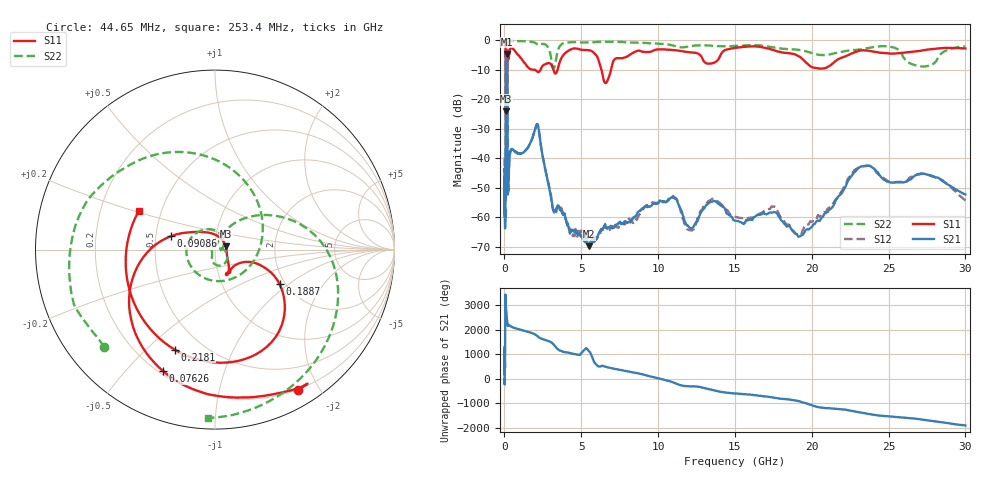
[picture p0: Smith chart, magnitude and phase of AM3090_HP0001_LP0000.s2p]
! Date/Time: Thu, Feb 28, 2019 1:53 PM
! Network Analyzer: Agilent Technologies E8364B Rev: A.07.50.67
! Sweep from 0.010 to 30.000 GHz, 1601 Points, Sweep Type: LOG
! Power Supply: 5.023 V, 0.002 A
# Hz S DB R 50
!freq MagS11 AngS11 MagS21 AngS21 MagS12 AngS12 MagS22 AngS22
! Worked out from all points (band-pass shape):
!   1601 points, 10 MHz to 30 GHz, reference 50 ohm
!   highest |S21| = -4.73 dB at 134.2 MHz (marker M1); lowest = -69.9 dB at 5.501 GHz (marker M2)
!   |S21| within 3 dB of the highest: 98.46 MHz to 174.1 MHz (75.63 MHz wide, 55.5 % of centre)
!   lowest |S11| = -24.1 dB at 98.44 MHz (marker M3), VSWR 1.13, Z = 56.3 + j2 ohm
!   |S11| at or under -10 dB: 1.806 GHz to 2.35 GHz (544.7 MHz wide, 26.2 % of centre); 3.182 GHz to 3.46 GHz (278.2 MHz wide, 8.38 % of centre); 6.308 GHz to 6.937 GHz (628.7 MHz wide, 9.49 % of centre)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
!   |S22| runs from -36.2 to -0.1 dB; largest |S21 - S12| = 0.013
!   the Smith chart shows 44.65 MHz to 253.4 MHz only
!   S11 on the Smith chart (normalised r, x): 44.65 MHz: 0.19, -1.73; 76.26 MHz: 0.22, -0.64; 90.86 MHz: 0.60, +0.10; 188.7 MHz: 1.86, -0.87; 218.1 MHz: 0.35, -0.61; 253.4 MHz: 0.37, +0.21
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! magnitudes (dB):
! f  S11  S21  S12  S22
! 10 MHz  -0.2  -44.5  -39.8  -0.5
! 38.04 MHz  -0.5  -60.0  -59.1  -1.3
! 44.65 MHz  -0.8  -56.7  -58.5  -1.7
! 76.26 MHz  -2.7  -42.9  -43.3  -5.2
! 90.86 MHz  -11.8  -14.0  -14.0  -15.2
! 98.44 MHz  -24.1  -7.7  -7.7  -16.6
! 134.2 MHz  -16.6  -4.7  -4.7  -29.8
! 144.7 MHz  -16.3  -4.9  -4.9  -21.2
! 169.8 MHz  -15.2  -6.8  -6.8  -36.1
! 188.7 MHz  -7.8  -17.8  -17.7  -10.7
! 218.1 MHz  -4.4  -52.3  -51.5  -1.5
! 253.4 MHz  -6.5  -50.7  -50.2  -0.6
! 550.5 MHz  -3.0  -37.2  -37.1  -0.2
! 2.084 GHz  -10.5  -28.8  -28.7  -1.2
! 3.236 GHz  -10.9  -58.1  -58.5  -9.4
! 5.501 GHz  -3.5  -69.9  -67.4  -0.8
! 6.619 GHz  -14.5  -63.5  -63.3  -0.6
! 7.926 GHz  -5.7  -61.6  -60.8  -0.8
! 10.81 GHz  -3.3  -53.5  -53.1  -1.7
! 19.41 GHz  -6.5  -66.0  -64.5  -3.5
! 23.36 GHz  -3.5  -42.8  -42.7  -3.0
! 30 GHz  -2.8  -52.3  -54.3  -2.2
